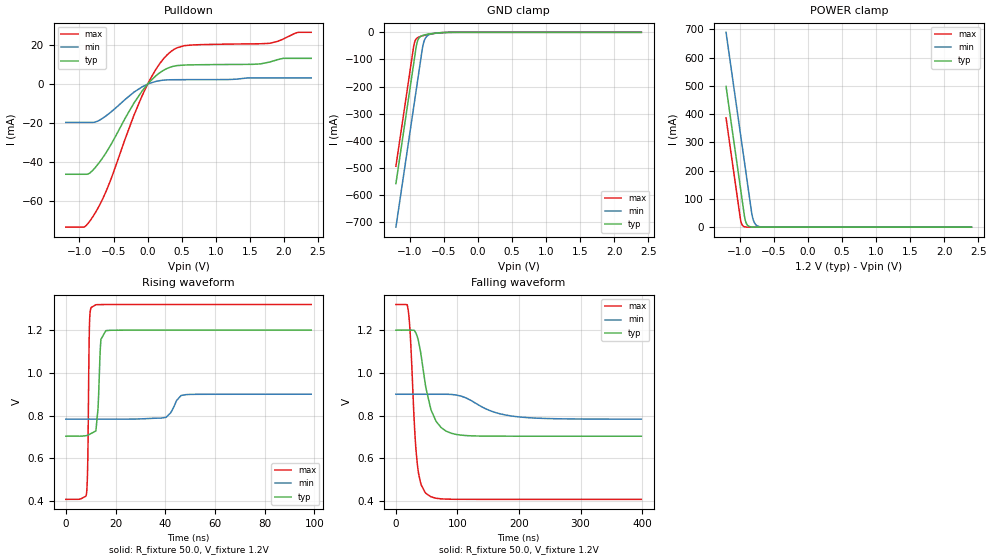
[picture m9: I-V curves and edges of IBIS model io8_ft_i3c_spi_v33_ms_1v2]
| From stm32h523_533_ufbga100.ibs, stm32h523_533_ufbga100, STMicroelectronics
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[Model]   io8_ft_i3c_spi_v33_ms_1v2
Model_type I/O_open_drain
Polarity   Non-Inverting
Enable   Active-Low
| CAP_THRESHOLD on pad IOFT is "UDTCAPC" :
| Rising=20.0% of vddiom   Falling=80.0% of vddiom
| C_comp min and max val. don't necessarily correlate with the min and max pvt
| but are the smallest and greatest pad capacitance found.
| var   typ   min   max
C_comp   3.39520pF  3.36985pF  3.42675pF
|C_comp_pulldown   3.39520pF  3.36985pF  3.42675pF
Vinl = 450.0mV
Vinh = 660.0mV
Vmeas = 600.0mV   | Reference voltage for timing measurements
Cref  = 50.0pF   | Timing specification test load capacitance value
Rref  = 1.0MOhm   | Timing specification test load resistance value
Vref  = 660.0mV   | Timing specification test load voltage
[Model Spec]
| TIME_THRESHOLD on pin ZII2CV11 is "CMOS" :
| Rising=40.0% of vdd   Falling=60.0% of vdd
Vinl 437.80000mV 335.80000mV 479.80000mV
Vinh 728.20000mV 529.20000mV 807.20000mV
| variable   typ   min   max
[Temperature Range] 25.0 125.0 -40.0
| variable   typ   min   max
[Voltage Range] 1.2V 900.0mV 1.32V
| variable   typ   min   max
[POWER Clamp Reference] 1.2V 900.0mV 1.32V
| variable   typ   min   max
[GND Clamp Reference] 0V 0V 0V
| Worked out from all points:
|   slope of the pulldown table from 0 to 0.18 V, typ, clamps not added: 30.6 ohm
|   GND clamp passes 1 mA (typ) near -0.52 V on its own axis
|   POWER clamp passes 1 mA (typ) near -0.84 V on its own axis
|   rising waveform, R_fixture 50.0, V_fixture 1.2V: 20-80 % time 1.11ns typ, 3.39ns min, 534ps max; typ from 0.704 V to 1.2 V
|   falling waveform, R_fixture 50.0, V_fixture 1.2V: 20-80 % time 20.8ns typ, 53.5ns min, 10.1ns max; typ from 1.2 V to 0.704 V
[POWER Clamp]
-1.2V     497.8mA    689.2mA    386.5mA
-990mV    140.8mA    332.2mA    29.53mA
-980mV    123.8mA    315.2mA    17.95mA
-960mV    89.81mA    281.2mA    6.634mA
-930mV    38.81mA    230.2mA    1.49mA
-900mV    12.07mA    179.2mA    334.8uA
-870mV    3.756mA    128.2mA    75.22uA
-820mV    536.4uA    44.98mA    6.246uA
-790mV    166.9uA    18.76mA    1.403uA
-750mV    35.18uA    5.846mA    191.8nA
-590mV    70.09nA    55uA       165.5pA
2.4V      0A         0A         0A
[GND Clamp]
-1.2V     -558.2mA   -719mA     -494.1mA
-940mV    -116.2mA   -277mA     -52.06mA
-930mV    -99.19mA   -260mA     -39.94mA
-900mV    -49.1mA    -209mA     -23.76mA
-880mV    -30.14mA   -175mA     -19.6mA
-850mV    -17.82mA   -124mA     -16.09mA
-810mV    -11.73mA   -56.78mA   -12.91mA
-780mV    -9.444mA   -28.21mA   -10.92mA
-740mV    -7.291mA   -13.16mA   -8.574mA
-640mV    -3.573mA   -4.171mA   -3.954mA
-380mV    -61.75uA   -230.3uA   -20.32uA
2.4V      3.863nA    718.4nA    150.6pA
| variable   typ   min   max
[Pullup Reference] 1.2V 900.0mV 1.32V
| variable   typ   min   max
[Pulldown Reference] 0V 0V 0V
[Pulldown]
-1.2V     -46.17mA   -19.62mA   -73.27mA
-930mV    -46.17mA   -19.62mA   -73.18mA
-770mV    -42.8mA    -19.41mA   -66.04mA
-570mV    -32.88mA   -15.18mA   -51.58mA
-200mV    -9.658mA   -4.083mA   -15.89mA
-80mV     -3.488mA   -1.363mA   -5.887mA
120mV     4.232mA    1.387mA    7.501mA
340mV     8.782mA    2.251mA    16.66mA
540mV     9.805mA    2.305mA    19.74mA
1.79V     11.33mA    3.206mA    20.93mA
2.2V      13.23mA    3.206mA    26.48mA
2.4V      13.23mA    3.206mA    26.56mA
[Ramp]
dV/dt_r 297.79756mV/1.03176ns 69.89566mV/3.07669ns 547.13369mV/532.60178ps
dV/dt_f 297.80513mV/20.20271ns 69.89173mV/53.15115ns 547.13934mV/10.02472ns
R_load = 50.0
| Removed startup time: 0s 0s 0s  .
| Removed end time: 98.75ns.
[Rising Waveform]
R_fixture   = 50.0
V_fixture   = 1.2V
V_fixture_min = 900.0mV
V_fixture_max = 1.32V
0s        703.7mV    783.5mV    408.1mV
8.3ns     706.3mV    783.5mV    431.8mV
8.85ns    708.6mV    783.5mV    592.8mV
9.5ns     712.1mV    783.5mV    1.212V
10.1ns    715.8mV    783.5mV    1.305V
12.1ns    728.2mV    783.5mV    1.319V
12.95ns   830mV      783.5mV    1.319V
14.15ns   1.157V     783.5mV    1.32V
16.15ns   1.198V     783.5mV    1.32V
98.75ns   1.2V       900mV      1.32V
| Removed startup time: 0s 0s 0s  .
| Removed end time: 398.75ns.
[Falling Waveform]
R_fixture   = 50.0
V_fixture   = 1.2V
V_fixture_min = 900.0mV
V_fixture_max = 1.32V
0s        1.2V       900mV      1.32V
19.85ns   1.2V       900mV      1.296V
23.15ns   1.2V       900mV      1.186V
30.4ns    1.197V     900mV      737.1mV
34.7ns    1.17V      900mV      574.1mV
48.85ns   927.6mV    900mV      435.8mV
65.1ns    773.9mV    900mV      413.2mV
97.65ns   712mV      896.6mV    408.3mV
191.7ns   703.7mV    796.7mV    408.1mV
398.8ns   703.7mV    783.5mV    408.1mV
